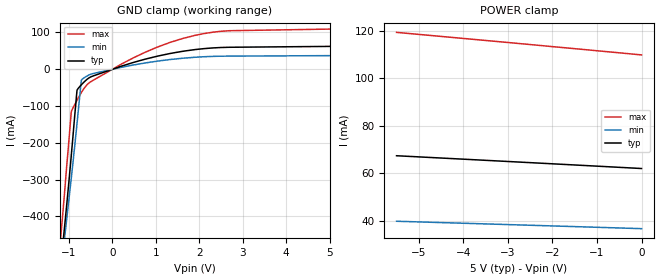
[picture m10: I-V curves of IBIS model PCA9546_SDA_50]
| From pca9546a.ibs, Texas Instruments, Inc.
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[Model]   PCA9546_SDA_50
Model_type  Terminator
| variable   typ   min   max
C_comp   6.44pF   5.08pF   8.31pF
| C_tri-state   6.44pF   5.08pF   8.31pF
[Temperature Range]   40   100   -40
| Ambient temperature   25   85   -40
[Voltage range]   5   4.5   5.5
[GND Clamp]
| PCA9546_SDA_50
|   Voltage   I(typ)   I(min)   I(max)
-5.5V     -4.176A    -3.989A    -4.398A
-1.2V     -545.3mA   -558.4mA   -473.9mA
-1.155V   -494.1mA   -514.2mA   -413.8mA
-1.11V    -441.7mA   -469.3mA   -351.4mA
-1.08V    -406mA     -438.9mA   -308.4mA
-945mV    -235.9mA   -297.1mA   -116.6mA
-810mV    -56.46mA   -145.3mA   -83.95mA
-710mV    -41.97mA   -29.19mA   -62.89mA
-620mV    -31.33mA   -21.05mA   -47.4mA
760mV     27.45mA    17.11mA    46.31mA
1.9V      53.3mA     32.48mA    91.88mA
5V        62.01mA    36.94mA    109mA
[POWER Clamp]
| PCA9546_SDA_50
|   Voltage   I(typ)   I(min)   I(max)
-5.5V     67.39mA    39.77mA    119.4mA
-2.79V    64.77mA    38.25mA    114.8mA
-1.16V    63.16mA    37.32mA    111.9mA
-95.1fV   62.01mA    36.65mA    109.9mA
